[IBIS Ver]   3.2
[Comment Char]   |_char
[File Name]   sprm448.ibs
[File Rev]   1.0
[Date]   November 15, 2006
[Source]   From Ansoft Q3D ver 7.0 result.
[Notes]
[Disclaimer]
[Copyright]
[Component]   c2801pz
[Manufacturer]   ti
[Package]
| variable   typ   min   max
R_pkg   2.03359e-001  1.85676e-001  2.33646e-001
L_pkg   4.42275e-009  3.91388e-009  5.16902e-009
C_pkg   6.90400e-013  6.03899e-013  7.98201e-013
[Pin]  signal_name   model_name   R_pin   L_pin   C_pin
01   GPIO12   BC3350ASHYPU   2.16292E-01  4.84246E-09  7.01525E-13
02   VSS   NC   2.05669E-01  4.59853E-09  7.81026E-13
03   VDDIO   NC   2.14427E-01  4.64717E-09  7.53822E-13
04   GPIO29   BC3325CSHYPU   2.26264E-01  4.68911E-09  7.55451E-13
05   GPIO33   BC3350ASHYPU   2.15510E-01  4.52774E-09  7.45637E-13
06   GPIO30   BC3325CSHYPU   2.05271E-01  4.36673E-09  7.14612E-13
07   GPIO31   BC3325CSHYPU   2.01452E-01  4.28833E-09  6.88677E-13
08   GPIO14   BC3350ASHYPU   1.93969E-01  4.17968E-09  6.67444E-13
09   GPIO15   BC3350ASHYPU   1.92673E-01  4.14893E-09  6.50213E-13
10   VDD   NC   1.88856E-01  4.10765E-09  6.26914E-13
11   VSS   NC   1.92989E-01  4.13681E-09  6.03899E-13
12   VDD1A18   NC   2.13333E-01  4.32411E-09  6.20891E-13
13   VSS1AGND   NC   2.06448E-01  4.25241E-09  6.31248E-13
14   VSSA2   NC   2.00063E-01  4.20609E-09  6.23019E-13
15   VDDA2   NC   1.93798E-01  4.16585E-09  6.28937E-13
16   ADCINA7   NC   1.89234E-01  4.18448E-09  6.36262E-13
17   ADCINA6   NC   1.87412E-01  4.23464E-09  6.46472E-13
18   ADCINA5   NC   1.86137E-01  4.27562E-09  6.59873E-13
19   ADCINA4   NC   1.85769E-01  4.34569E-09  6.75681E-13
20   ADCINA3   NC   1.87173E-01  4.42449E-09  6.94435E-13
21   ADCINA2   NC   1.89523E-01  4.53444E-09  7.11496E-13
22   ADCINA1   NC   1.93470E-01  4.65439E-09  7.32914E-13
23   ADCINA0   NC   1.96936E-01  4.78656E-09  7.54045E-13
24   ADCLO   NC   2.02141E-01  4.91416E-09  7.75388E-13
25   VSSAIO   NC   2.06429E-01  5.12034E-09  6.92931E-13
26   VDDAIO   NC   2.05491E-01  4.95382E-09  6.92435E-13
27   ADCINB0   NC   2.00858E-01  4.71178E-09  7.76728E-13
28   ADCINB1   NC   1.94857E-01  4.55615E-09  7.54959E-13
29   ADCINB2   NC   1.92781E-01  4.41548E-09  7.34283E-13
30   ADCINB3   NC   1.88419E-01  4.26915E-09  7.14862E-13
31   ADCINB4   NC   1.86413E-01  4.13080E-09  6.95435E-13
32   ADCINB5   NC   1.85676E-01  4.05447E-09  6.78346E-13
33   ADCINB6   NC   1.86563E-01  3.97672E-09  6.63340E-13
34   ADCINB7   NC   1.88600E-01  3.93329E-09  6.49418E-13
35   ADCREFIN   NC   1.91978E-01  3.91388E-09  6.38953E-13
36   ADCREFM   NC   1.97273E-01  3.93821E-09  6.32494E-13
37   ADCREFP   NC   2.04030E-01  4.00314E-09  6.29101E-13
38   ADCRESEXT   NC   2.12412E-01  4.05794E-09  6.41591E-13
39   VSS2AGND   NC   2.20295E-01  4.17640E-09  6.49431E-13
40   VDD2A18   NC   2.26915E-01  4.30270E-09  6.53434E-13
41   VSS   NC   2.25777E-01  4.36227E-09  6.44913E-13
42   VDD   NC   2.09612E-01  4.25306E-09  6.56261E-13
43   GPIO34   BC3350ASHYPU   2.17167E-01  4.40172E-09  6.83134E-13
44   GPIO1   BC3350ASHYPU   2.19379E-01  4.51534E-09  6.94421E-13
45   GPIO2   BC3350ASHYPU   2.16721E-01  4.56076E-09  7.15544E-13
46   VDDIO   NC   2.26017E-01  4.78354E-09  7.35852E-13
47   GPIO0   BC3350ASHYPU   2.11005E-01  4.69198E-09  7.46315E-13
48   GPIO3   BC3350ASHYPU   2.21106E-01  4.92036E-09  7.83494E-13
49   VSS   NC   2.33646E-01  5.16902E-09  7.98201E-13
50   GPIO16   BC3350ASHYPU   2.13744E-01  5.12910E-09  6.84259E-13
51   GPIO4   BC3350ASHYPU   2.26398E-01  4.92342E-09  7.06407E-13
52   GPIO17   BC3350ASHYPU   2.15844E-01  4.68935E-09  7.95814E-13
53   GPIO5   BC3350ASHYPU   2.04033E-01  4.50014E-09  7.72035E-13
54   GPIO18   BC3350ASHYPU   1.95635E-01  4.36218E-09  7.46249E-13
55   VSS   NC   1.89527E-01  4.27092E-09  7.11302E-13
56   GPIO6   BC3350ASHYPU   1.96559E-01  4.26988E-09  6.97016E-13
57   GPIO19   BC3350ASHYPU   1.91406E-01  4.17811E-09  6.85500E-13
58   GPIO7   BC3350ASHYPU   1.87512E-01  4.10710E-09  6.64382E-13
59   VDD   NC   1.85845E-01  4.07460E-09  6.37606E-13
60   GPIO8   BC3350ASHYPU   1.88779E-01  4.07856E-09  6.23034E-13
61   GPIO9   BC3350ASHYPU   1.86926E-01  4.03716E-09  6.20859E-13
62   VSS   NC   1.86440E-01  4.04566E-09  6.02703E-13
63   GPIO20   BC3350ASHYPU   1.88373E-01  4.05495E-09  6.04095E-13
64   GPIO10   BC3350ASHYPU   1.88009E-01  4.08425E-09  6.12057E-13
65   VDDIO   NC   1.85978E-01  4.10911E-09  6.20487E-13
66   XCLKOUT   BC3325CSFSHY   1.86925E-01  4.17194E-09  6.25512E-13
67   GPIO21   BC3350ASHYPU   1.86819E-01  4.21956E-09  6.40861E-13
68   VDD   NC   1.89866E-01  4.31866E-09  6.54786E-13
69   VSS   NC   1.85610E-01  4.34307E-09  6.58781E-13
70   GPIO11   BC3350ASHYPU   1.86090E-01  4.36372E-09  6.88671E-13
71   GPIO22   BC3350ASHYPU   1.86568E-01  4.45206E-09  7.16155E-13
72   GPIO23   BC3350ASHYPU   1.87669E-01  4.56253E-09  7.38219E-13
73   TDI   IC33SFSHYPU   1.93987E-01  4.72336E-09  7.60132E-13
74   TMS   IC33SFSHYPU   2.01048E-01  4.88251E-09  7.86418E-13
75   TCK   IC33SFSHYPU   2.11249E-01  5.18088E-09  7.03348E-13
76   TDO   OC3325CS   2.06688E-01  4.94914E-09  6.96076E-13
77   VSS   NC   1.98342E-01  4.65382E-09  7.80676E-13
78   XRSn   BC3350BTODHYPU   1.93176E-01  4.48692E-09  7.57321E-13
79   GPIO27   BC3350ASHYPU   1.88188E-01  4.31589E-09  7.28548E-13
80   EMU0   BC3325CSHYPU   1.89619E-01  4.26207E-09  7.10142E-13
81   EMU1   BC3325CSHYPU   1.86922E-01  4.12139E-09  6.97582E-13
82   VDDIO   NC   1.85269E-01  4.01949E-09  6.82524E-13
83   GPIO24   BC3350ASHYPU   1.85832E-01  3.93920E-09  6.64624E-13
84   TRSTn   IC33SFSHYPD   1.87384E-01  3.90020E-09  6.46879E-13
85   VDD   NC   1.90176E-01  3.87909E-09  6.26008E-13
86   X2   NC   1.85448E-01  3.83198E-09  6.08398E-13
87   VSS   NC   1.87288E-01  3.82154E-09  6.08983E-13
88   X1   NC   1.89799E-01  3.81436E-09  6.13885E-13
89   VSS   NC   1.91602E-01  3.87476E-09  6.15372E-13
90   XCLKIN   BC3350ASHYPU   1.95306E-01  3.94123E-09  6.27780E-13
91   GPIO25   BC3350ASHYPU   1.99443E-01  4.04240E-09  6.37161E-13
92   GPIO28   BC3325CSHYPU   2.03022E-01  4.16398E-09  6.48097E-13
93   VDD   NC   2.00114E-01  4.20193E-09  6.56967E-13
94   VSS   NC   1.90892E-01  4.16295E-09  6.61041E-13
95   GPIO13   BC3350ASHYPU   1.86615E-01  4.16393E-09  6.81384E-13
96   VDDIO   NC   1.84802E-01  4.25057E-09  7.10450E-13
99   GPIO26   BC3350ASHYPU   1.97169E-01  4.74011E-09  7.77284E-13
100   GPIO32   BC3350ASHYPU   2.04213E-01  5.01635E-09  6.90838E-13
[Define Package Model]  pz_agni_1
[Manufacturer]   ti
[OEM]   xyz
[Description]  None
[Number Of Pins]  100
[Pin Numbers]
01   | 01 = P001
02   | 02 = P002
03   | 03 = P003
04   | 04 = P004
05   | 05 = P005
06   | 06 = P006
07   | 07 = P007
08   | 08 = P008
09   | 09 = P009
10   | 10 = P010
11   | 11 = P011
12   | 12 = P012
13   | 13 = P013
14   | 14 = P014
15   | 15 = P015
16   | 16 = P016
17   | 17 = P017
18   | 18 = P018
19   | 19 = P019
20   | 20 = P020
21   | 21 = P021
22   | 22 = P022
23   | 23 = P023
24   | 24 = P024
25   | 25 = P025
26   | 26 = P026
27   | 27 = P027
28   | 28 = P028
29   | 29 = P029
30   | 30 = P030
31   | 31 = P031
32   | 32 = P032
33   | 33 = P033
34   | 34 = P034
35   | 35 = P035
36   | 36 = P036
37   | 37 = P037
38   | 38 = P038
39   | 39 = P039
40   | 40 = P040
41   | 41 = P041
42   | 42 = P042
43   | 43 = P043
44   | 44 = P044
45   | 45 = P045
46   | 46 = P046
47   | 47 = P047
48   | 48 = P048
49   | 49 = P049
50   | 50 = P050
51   | 51 = P051
52   | 52 = P052
53   | 53 = P053
54   | 54 = P054
55   | 55 = P055
56   | 56 = P056
57   | 57 = P057
58   | 58 = P058
59   | 59 = P059
60   | 60 = P060
61   | 61 = P061
62   | 62 = P062
63   | 63 = P063
64   | 64 = P064
65   | 65 = P065
66   | 66 = P066
67   | 67 = P067
68   | 68 = P068
69   | 69 = P069
70   | 70 = P070
71   | 71 = P071
72   | 72 = P072
73   | 73 = P073
74   | 74 = P074
75   | 75 = P075
76   | 76 = P076
77   | 77 = P077
78   | 78 = P078
79   | 79 = P079
80   | 80 = P080
81   | 81 = P081
82   | 82 = P082
83   | 83 = P083
84   | 84 = P084
85   | 85 = P085
86   | 86 = P086
87   | 87 = P087
88   | 88 = P088
89   | 89 = P089
90   | 90 = P090
91   | 91 = P091
92   | 92 = P092
93   | 93 = P093
94   | 94 = P094
95   | 95 = P095
96   | 96 = P096
97   | 97 = P097
98   | 98 = P098
99   | 99 = P099
100   | 100 = P100
[Model Data]
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[End Model Data]
[End Package Model]
|   Component BC3325CSFSHY
[Component]   BC3325CSFSHY
[Manufacturer]   Texas Instruments
[Package]
|  variable   typ   min   max
R_pkg   0   0   0
L_pkg   0   0   0
C_pkg   0   0   0
[Pin]   signal_name   model_name   R_pin   L_pin   C_pin
VSS   VSS   GND
VDDS   VDDS   POWER
PAD   PAD   BC3325CSFSHY
|   Component OC3325CS
[Component]   OC3325CS
[Manufacturer]   Texas Instruments
[Package]
|  variable   typ   min   max
R_pkg   0   0   0
L_pkg   0   0   0
C_pkg   0   0   0
[Pin]   signal_name   model_name   R_pin   L_pin   C_pin
VSS   VSS   GND
VDDS   VDDS   POWER
PAD   PAD   OC3325CS
|   Component IDH091_OUJ431
[Component]   IDH091_OUJ431
[Manufacturer]   Texas Instruments
[Package]
|  variable   typ   min   max
R_pkg   0   0   0
L_pkg   0   0   0
C_pkg   0   0   0
[Pin]   signal_name   model_name   R_pin   L_pin   C_pin
VSS   VSS   GND
VDDS   VDDS   POWER
PAD   PAD   IDH091_OUJ431
|   Component IC33SFSHYPD
[Component]   IC33SFSHYPD
[Manufacturer]   Texas Instruments
[Package]
|  variable   typ   min   max
R_pkg   0   0   0
L_pkg   0   0   0
C_pkg   0   0   0
[Pin]   signal_name   model_name   R_pin   L_pin   C_pin
VSS   VSS   GND
VDDS   VDDS   POWER
PAD   PAD   IC33SFSHYPD
[Model Selector] IC33SFSHYPD
PULLDOWN_ON_3P3_1  Cell operated at 3.3(nom)
|BUFFER OPERATING IN WEAK PULLDOWN MODE
PULLDOWN_OFF_3P3_1  Cell operated at 3.3(nom)
|   Component IC33SFSHY
[Component]   IC33SFSHY
[Manufacturer]   Texas Instruments
[Package]
|  variable   typ   min   max
R_pkg   0   0   0
L_pkg   0   0   0
C_pkg   0   0   0
[Pin]   signal_name   model_name   R_pin   L_pin   C_pin
VSS   VSS   GND
VDDS   VDDS   POWER
PAD   PAD   IC33SFSHY
|   Component BC3350ASHYPU
[Component]   BC3350ASHYPU
[Manufacturer]   Texas Instruments
[Package]
|  variable   typ   min   max
R_pkg   0   0   0
L_pkg   0   0   0
C_pkg   0   0   0
[Pin]   signal_name   model_name   R_pin   L_pin   C_pin
VSS   VSS   GND
VDDS   VDDS   POWER
PAD   PAD   BC3350ASHYPU
[Model Selector] BC3350ASHYPU
PULLUP_ON_3P3_2  Cell operated at 3.3(nom)
|BUFFER OPERATING IN WEAK PULLUP MODE
PULLUP_OFF_3P3_2  Cell operated at 3.3(nom)
|   Component BC3325CSHYPU
[Component]   BC3325CSHYPU
[Manufacturer]   Texas Instruments
[Package]
|  variable   typ   min   max
R_pkg   0   0   0
L_pkg   0   0   0
C_pkg   0   0   0
[Pin]   signal_name   model_name   R_pin   L_pin   C_pin
VSS   VSS   GND
VDDS   VDDS   POWER
PAD   PAD   BC3325CSHYPU
[Model Selector] BC3325CSHYPU
PULLUP_ON_3P3_3  Cell operated at 3.3(nom)
|BUFFER OPERATING IN WEAK PULLUP MODE
PULLUP_OFF_3P3_3  Cell operated at 3.3(nom)
|   Component OUJ431
[Component]   OUJ431
[Manufacturer]   Texas Instruments
[Package]
|  variable   typ   min   max
R_pkg   0   0   0
L_pkg   0   0   0
C_pkg   0   0   0
[Pin]   signal_name   model_name   R_pin   L_pin   C_pin
VSS   VSS   GND
VDDS   VDDS   POWER
PAD   PAD   OUJ431
|   Component IC33SFSHYPU
[Component]   IC33SFSHYPU
[Manufacturer]   Texas Instruments
[Package]
|  variable   typ   min   max
R_pkg   0   0   0
L_pkg   0   0   0
C_pkg   0   0   0
[Pin]   signal_name   model_name   R_pin   L_pin   C_pin
VSS   VSS   GND
VDDS   VDDS   POWER
PAD   PAD   IC33SFSHYPU
[Model Selector] IC33SFSHYPU
PULLUP_ON_3P3_4  Cell operated at 3.3(nom)
|BUFFER OPERATING IN WEAK PULLUP MODE
PULLUP_OFF_3P3_4  Cell operated at 3.3(nom)
|   Component BC3350BTODHYPU
[Component]   BC3350BTODHYPU
[Manufacturer]   Texas Instruments
[Package]
|  variable   typ   min   max
R_pkg   0   0   0
L_pkg   0   0   0
C_pkg   0   0   0
[Pin]   signal_name   model_name   R_pin   L_pin   C_pin
VSS   VSS   GND
VDDS   VDDS   POWER
PAD   PAD   BC3350BTODHYPU
| Models and submodels in the file (14): BC3325CSFSHY (I/O), OC3325CS (3-state), IDH091_OUJ431 (I/O), PULLDOWN_ON_3P3_1 (Input), PULLDOWN_OFF_3P3_1 (Input), IC33SFSHY (Input), PULLUP_ON_3P3_2 (I/O), PULLUP_OFF_3P3_2 (I/O), PULLUP_ON_3P3_3 (I/O), PULLUP_OFF_3P3_3 (I/O), OUJ431 (3-state), PULLUP_ON_3P3_4 (Input), PULLUP_OFF_3P3_4 (Input), BC3350BTODHYPU (I/O_open_drain)
